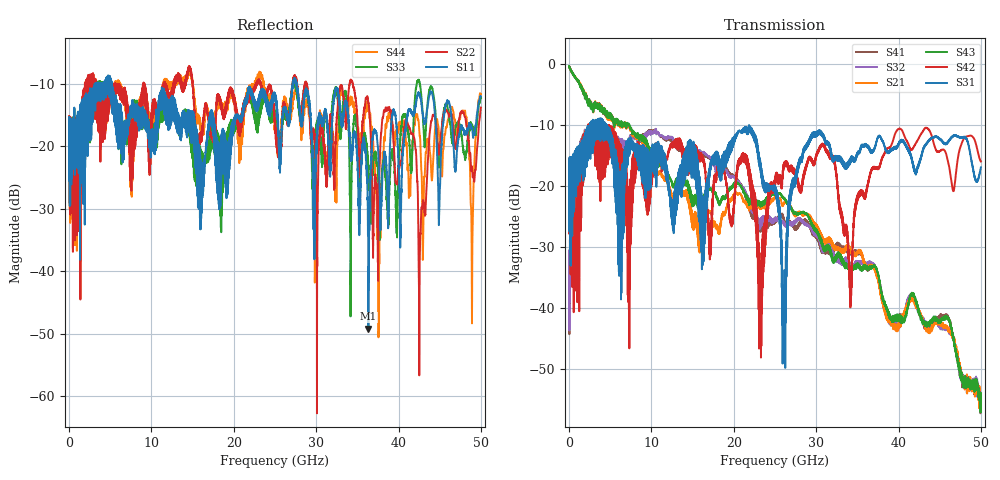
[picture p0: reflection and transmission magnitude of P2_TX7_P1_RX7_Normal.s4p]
!Keysight Technologies,N5225A,MY51441389,A.10.49.11
!Date: Monday, July 08, 2019 15:01:31
!Correction: S11(Full 4 Port(1,2,3,4))
!S12(Full 4 Port(1,2,3,4))
!S13(Full 4 Port(1,2,3,4))
!S14(Full 4 Port(1,2,3,4))
!S21(Full 4 Port(1,2,3,4))
!S22(Full 4 Port(1,2,3,4))
!S23(Full 4 Port(1,2,3,4))
!S24(Full 4 Port(1,2,3,4))
!S31(Full 4 Port(1,2,3,4))
!S32(Full 4 Port(1,2,3,4))
!S33(Full 4 Port(1,2,3,4))
!S34(Full 4 Port(1,2,3,4))
!S41(Full 4 Port(1,2,3,4))
!S42(Full 4 Port(1,2,3,4))
!S43(Full 4 Port(1,2,3,4))
!S44(Full 4 Port(1,2,3,4))
!S4P File: Measurements: <S11,S12,S13,S14>,
!<S21,S22,S23,S24>,
!<S31,S32,S33,S34>,
!<S41,S42,S43,S44>:
# Hz S  dB  R 50
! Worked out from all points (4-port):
!   5000 points, 10 MHz to 50 GHz, reference 50 ohm
!   strongest paths, dB at 10 MHz, 12.51 GHz, 25.01 GHz, 37.51 GHz, 50 GHz:
!     S31: -19.4, -26.4, -20.0, -12.1, -17.0
!     S42: -19.4, -13.3, -18.7, -17.2, -16.0
!     S43: -0.4, -19.8, -21.5, -34.5, -57.1
!     S21: -0.4, -22.4, -21.8, -35.5, -54.9
!     S32: -33.1, -12.0, -25.5, -34.5, -55.9
!     S41: -33.0, -12.3, -25.7, -35.1, -55.5
!   lowest |S11| = -49.2 dB at 36.34 GHz (marker M1), VSWR 1.01, Z = 50.1 - j0.339 ohm
!   |S11| at or under -10 dB: start of sweep to 3.11 GHz; 5.201 GHz to 27.14 GHz (21.94 GHz wide, 136 % of centre); 27.64 GHz to end of sweep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
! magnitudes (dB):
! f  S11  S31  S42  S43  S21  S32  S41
! 10 MHz  -17.8  -19.4  -19.4  -0.4  -0.4  -33.1  -33.0
! 2.12 GHz  -13.4  -11.7  -12.1  -5.9  -5.8  -11.3  -11.2
! 22.01 GHz  -11.3  -10.4  -17.9  -22.9  -23.6  -23.2  -24.1
! 26.1 GHz  -13.8  -41.8  -16.2  -22.2  -22.9  -26.4  -25.8
! 36.34 GHz  -49.2  -13.7  -19.5  -33.4  -33.2  -32.5  -33.4
! 42.63 GHz  -12.1  -15.8  -11.8  -41.1  -41.0  -41.1  -40.9
! 50 GHz  -12.1  -17.0  -16.0  -57.1  -54.9  -55.9  -55.5
